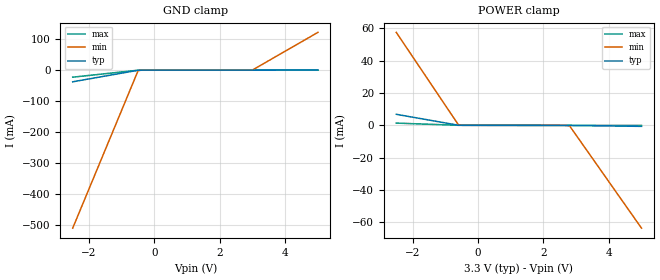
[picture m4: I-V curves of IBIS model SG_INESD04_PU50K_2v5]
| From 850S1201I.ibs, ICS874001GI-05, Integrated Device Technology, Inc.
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[Model] SG_INESD04_PU50K_2v5
Model_type   Input
Polarity   Non-Inverting
Vinl = 0.70V
Vinh = 1.7V
|   typ   min   max
C_comp   2pF   1.5pF   2.5pF
|   typ   min   max
[Voltage range]  3.3V   3.15V   3.45V
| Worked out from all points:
|   GND clamp passes 1 mA (typ) near -0.53 V on its own axis
|   POWER clamp passes 1 mA (typ) near -0.87 V on its own axis
[GND_clamp]
|Voltage   I(typ)   I(min)   I(max)
-2.5V     -37.48mA   -508.7mA   -22.63mA
-500mV    -417.9uA   -1.694mA   -206.2uA
3V        12.83uA    572.1uA    7.099uA
5V        824.4uA    121.6mA    45.97uA
[POWER_clamp]
|Voltage   I(typ)   I(min)   I(max)
-2.5V     6.822mA    57.58mA    1.373mA
-600mV    53.4uA     339.2uA    15.55uA
2.8V      -56.65uA   -309.7uA   -53.03uA
5V        -645.9uA   -63.69mA   -95.27uA
